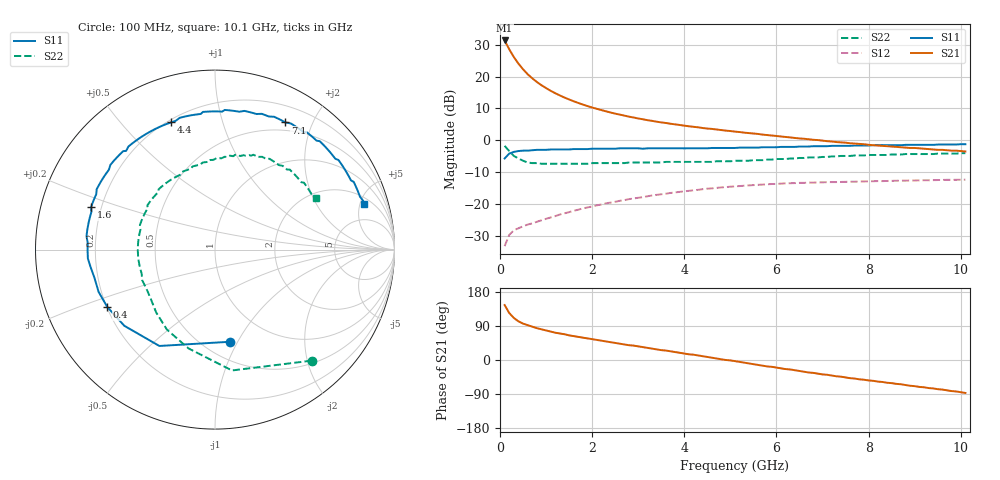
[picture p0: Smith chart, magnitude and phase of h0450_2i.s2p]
!HBFP-0450
!S and NOISE PARAMETERS at Vce=2V  Ic=70mA.  LAST UPDATED  09-04-98
# GHZ S MA R  50
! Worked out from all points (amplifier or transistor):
!   101 points, 100 MHz to 10.1 GHz, reference 50 ohm
!   highest |S21| = 31.3 dB at 100 MHz (marker M1)
!   |S21| within 3 dB of that: start of sweep to 210.5 MHz
!   unconditionally stable (mu >= 1): 2.087 GHz to end of sweep
!   at 1.7 GHz: K = 0.97, MSG = 16.7 dB, |S12| = -21.7 dB
!   at 5.1 GHz: K = 1.09, MAG = 6.7 dB, |S12| = -14.4 dB
!   at 10.1 GHz: K = 1.04, MAG = 3.1 dB, |S12| = -12.3 dB
!   lowest NFmin = 2.07 dB at 1.8 GHz
!   S11 on the Smith chart (normalised r, x): 100 MHz: 0.66, -0.93; 400 MHz: 0.20, -0.24; 1.6 GHz: 0.16, +0.16; 4.4 GHz: 0.21, +0.69; 7.1 GHz: 0.39, +1.63; 10.1 GHz: 2.62, +5.47
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0.1  0.52 -81.0  36.71 145.0  0.022 61.0  0.82 -49.0
0.2  0.62 -120.0  26.77 124.0  0.033 46.0  0.68 -82.0
0.3  0.66 -140.0  20.2 111.0  0.039 40.0  0.57 -105.0
0.4  0.68 -152.0  15.9 102.0  0.042 38.0  0.52 -121.0
0.5  0.69 -160.0  13 96.0  0.045 37.0  0.48 -133.0
0.6  0.69 -167.0  10.87 92.0  0.048 37.0  0.45 -143.0
0.7  0.7 -172.0  9.37 88.0  0.05 38.0  0.44 -150.0
0.8  0.71 -176.0  8.21 84.0  0.053 38.0  0.44 -157.0
0.9  0.71 -180.0  7.31 81.0  0.056 39.0  0.43 -162.0
1.1  0.72 174.0  5.97 75.0  0.062 39.0  0.43 -172.0
1.3  0.72 168.0  5.05 70.0  0.069 40.0  0.43 -179.0
1.6  0.73 161.0  4.09 63.0  0.079 39.0  0.43 172.0
1.8  0.73 157.0  3.63 59.0  0.086 38.0  0.43 167.0
2.1  0.74 151.0  3.12 53.0  0.096 36.0  0.44 160.0
2.5  0.74 143.0  2.62 45.0  0.109 33.0  0.44 152.0
3.5  0.75 125.0  1.91 26.0  0.143 23.0  0.45 135.0
4.4  0.75 109.0  1.56 10.0  0.172 11.0  0.46 119.0
5.1  0.76 96.0  1.37 -3.0  0.19 1.0  0.48 105.0
6.8  0.81 66.0  1.02 -34.0  0.218 -24.0  0.54 76.0
7.1  0.81 61.0  0.97 -39.0  0.221 -29.0  0.55 72.0
8.5  0.84 40.0  0.8 -61.0  0.232 -47.0  0.6 51.0
10.1  0.87 17.0  0.67 -87.0  0.242 -70.0  0.63 27.0
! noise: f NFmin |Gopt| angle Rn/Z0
1.8  2.07  0.64  -151  0.12
2  2.07  0.64  -148  0.14
2.5  2.21  0.66  -139  0.21
3.5  2.47  0.69  -122  0.43
4  2.61  0.71  -112  0.63
5  2.87  0.73  -94  1.08
5.5  3.01  0.75  -85  1.47
7  3.41  0.79  -59  2.88
8  3.67  0.81  -43  4.14
10  4.2  0.82  -15  6.48
